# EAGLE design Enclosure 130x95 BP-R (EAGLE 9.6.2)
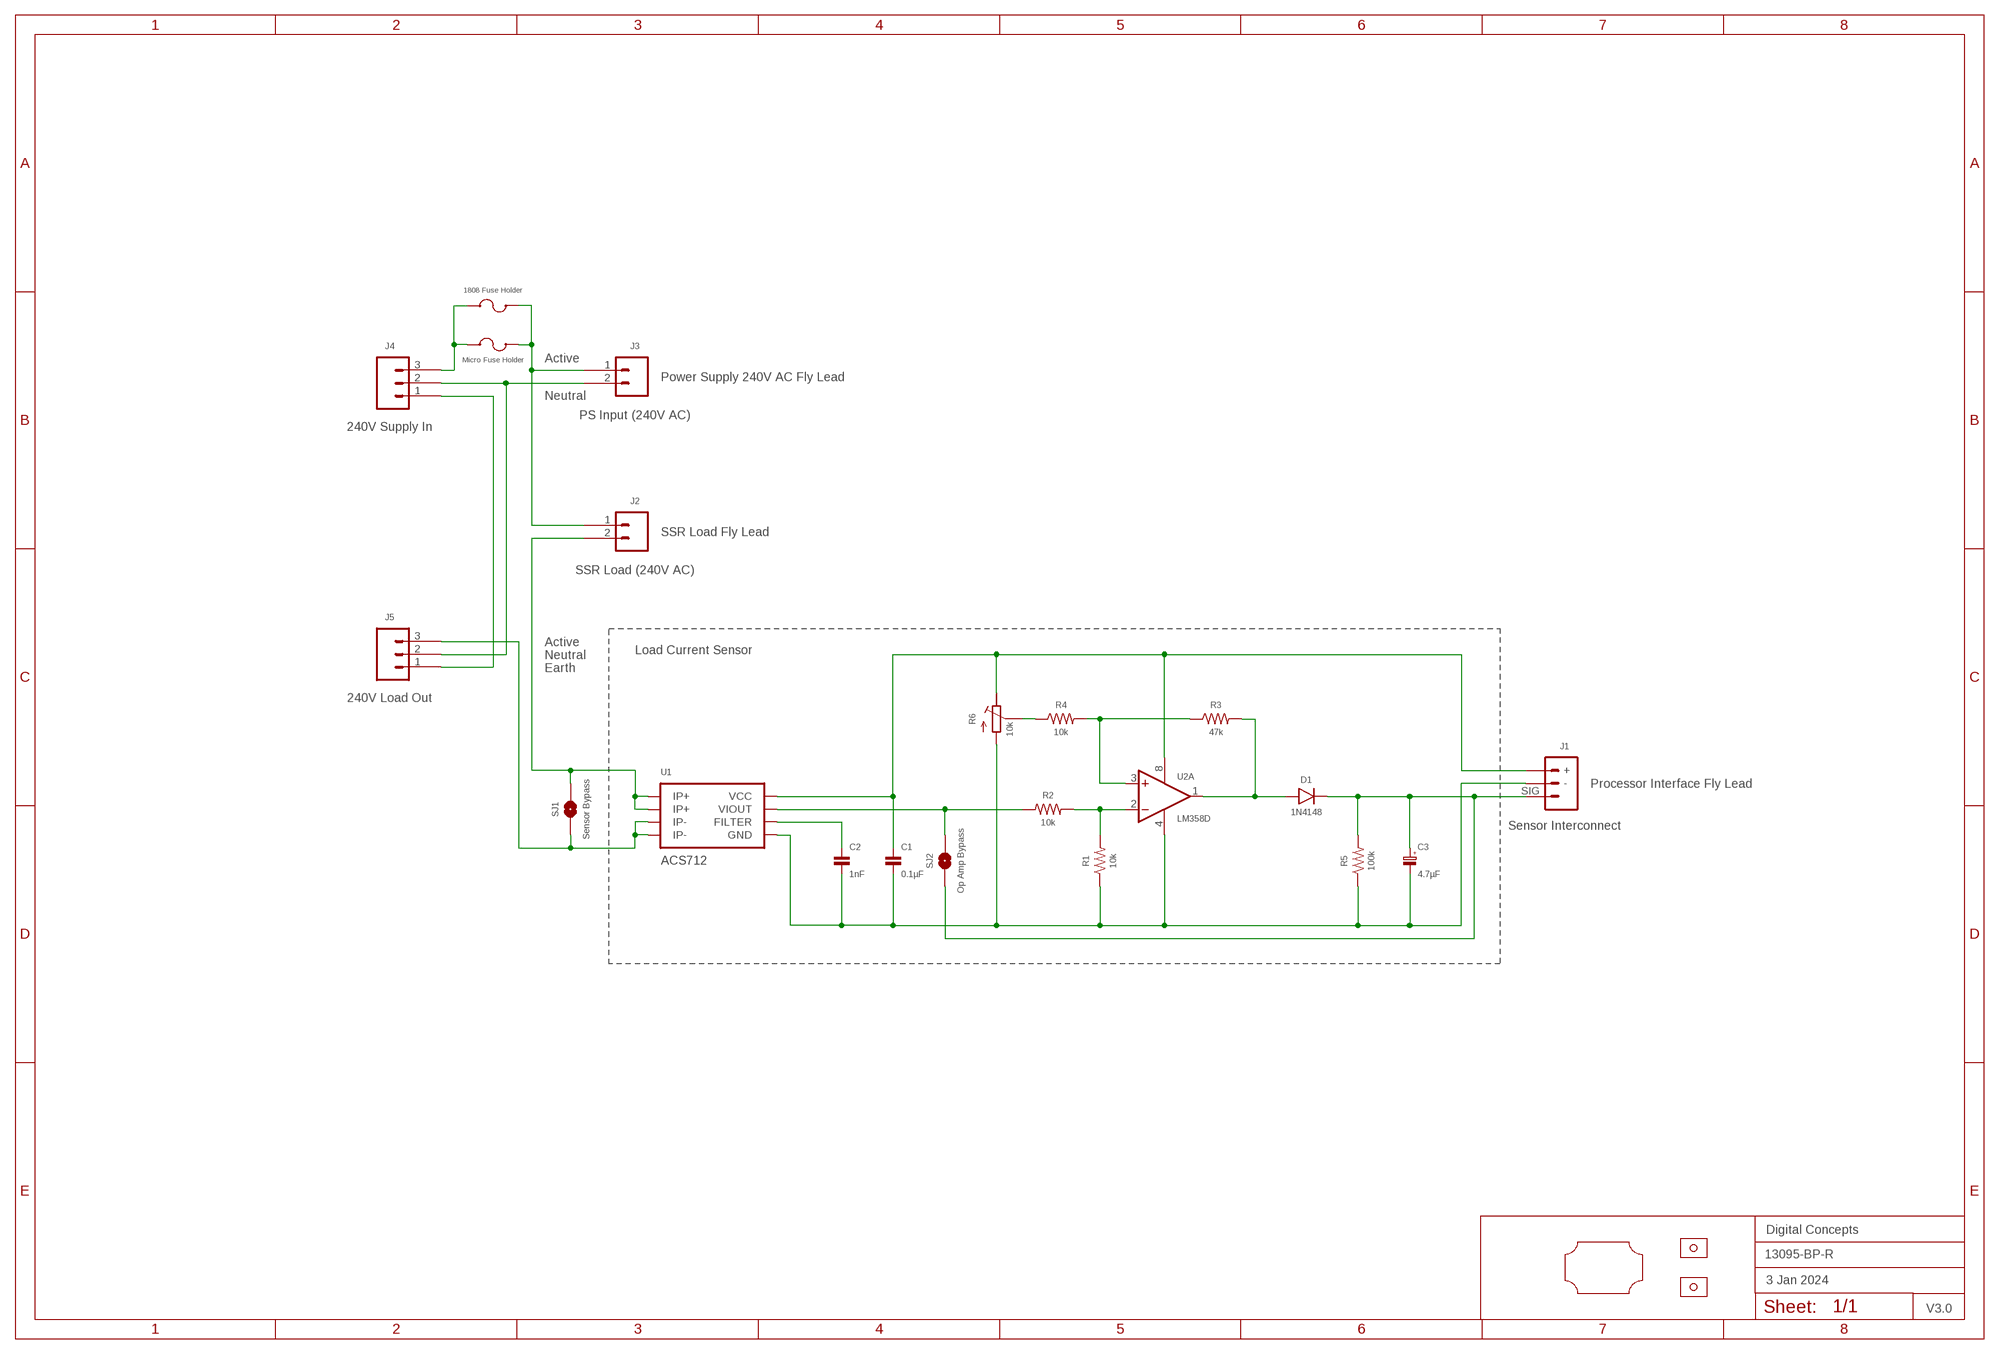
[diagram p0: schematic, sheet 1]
FRAME2 (A3L-LOC): DATE: 3 Jan 2024; OWNER: Digital Concepts; TITLE: 13095-BP-R; VERSION: V3.0

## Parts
C1  0.1µF  CAPACITOR-0805  [C0805]
C2  1nF  CAPACITOR-0805  [C0805]
C3  4.7µF  CAPACITOR-1206-TANTALUM  [C1206-POLARISED]
D1  1N4148  DIODE-1N4148-SOD323  [SOD-323]
F2  1808 Fuse Holder  FUSE-HOLDER-1808  [FUSE-HOLDER-1808]
J1  Sensor Interconnect  JST-PH2.0-3-HORIZONTAL  [JST-PH2.0-3-HORIZONTAL-SIG]
J2  SSR Load (240V AC)  TERMINAL_SCREW_2P_VERTICAL  [TERMINAL-SCREW-2P]
J3  PS Input (240V AC)  JST-XH2.54-2-HORIZONTAL  [JST-XH2.4-2-HORIZONTAL]
J4  240V Supply In  TERMINAL_SCREW_3P_VERTICAL  [TERMINAL-SCREW-3P]
J5  240V Load Out  TERMINAL_SCREW_3P_VERTICAL  [TERMINAL-SCREW-3P]
R1  10k  RESISTORR0805  [R0805]
R2  10k  RESISTORR0805  [R0805]
R3  47k  RESISTORR0805  [R0805]
R4  10k  RESISTORR0805  [R0805]
R5  100k  RESISTORR0805  [R0805]
R6  10k  RESISTOR-TRIMM-3386P  [RTRIM3386P]
SJ1  Sensor Bypass  SJ  [SJ]
SJ2  Op Amp Bypass  SJ  [SJ]
U1  ACS712  [SOP-8]
U2  LM358D  [SOP-8]
U$1  PCB-OUTLINE-130X95-MAX-RC-H3  [PROTO-130X95-OUTLINE-MAX-RC-H3]
U$2  Micro Fuse Holder  FUSE-HOLDER  [FUSE-HOLDER-MICRO]
U$4  STRAIN-RELIEF-SADDLE  [STRAIN-RELIEF-SADDLE]
U$5  STRAIN-RELIEF-SADDLE  [STRAIN-RELIEF-SADDLE]

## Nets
ACTIVE_IN: F2.P$2 J2.1 J3.1 U$2.P$3 U$2.P$4
ACTIVE_OUT: J2.2 SJ1.2 U1.1(IP+) U1.2(IP+)
EARTH: J4.1 J5.1
N$2: C1.1 J1.+ R6.1(E) U1.8(VCC) U2.8(P:V+)
N$3: C3.1(+) D1.C J1.SIG R5.2 SJ2.1
N$4: D1.A R3.2 U2.1(A:OUT)
N$5: R3.1 R4.2 U2.3(A:+IN)
N$6: R4.1 R6.2(S)
N$7: F2.P$1 J4.3 U$2.P$1 U$2.P$2
N$8: R1.2 R2.2 U2.2(A:-IN)
N$19: J5.3 SJ1.1 U1.3(IP-) U1.4(IP-)
N$20: C1.2 C2.2 C3.2(-) J1.- R1.1 R5.1 R6.3(A) U1.5(GND) U2.4(P:V-)
N$22: R2.1 SJ2.2 U1.7(VIOUT)
N$24: C2.1 U1.6(FILTER)
NEUTRAL: J3.2 J4.2 J5.2
Unconnected: U2.5(B:+IN) U2.6(B:-IN) U2.7(B:OUT)

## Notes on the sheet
- Active
- Power Supply 240V AC Fly Lead
- Neutral
- SSR Load Fly Lead
- Active
- Neutral | Load Current Sensor
- Earth
- Processor Interface Fly Lead

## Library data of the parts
C1 C2 = digitalconcepts:CAPACITOR-0805: 0805 Capacitor
C3 = digitalconcepts:CAPACITOR-1206-TANTALUM: Capacitor 1206 Tantalum
D1 = digitalconcepts:DIODE-1N4148-SOD323: 1N4148 SOD-323
F2 = digitalconcepts:FUSE-HOLDER-1808: 1808 Fuse Holder
J1 = digitalconcepts:JST-PH2.0-3-HORIZONTAL: PH2.0 3P Horizontal Connector
J2 = digitalconcepts:TERMINAL_SCREW_2P_VERTICAL: PCB Mount Screw-Type Terminal 2P
J3 = digitalconcepts:JST-XH2.54-2-HORIZONTAL: XH2.54 2P Horizontal Connector
J4 J5 = digitalconcepts:TERMINAL_SCREW_3P_VERTICAL: PCB Mount Screw-Type Terminal 3P
R1-R5 = digitalconcepts:RESISTOR: Resistor; SPICEPREFIX: R
R6 = digitalconcepts:RESISTOR-TRIMM-3386P: BOURNS Trim Pot 3386P
SJ1 SJ2 = digitalconcepts:SJ: Solder Jumper
U1 = digitalconcepts:ACS712: ACS712 Hall-Effect-Based Linear Current Sensor IC
U2 = digitalconcepts:LM358: OP AMP also LM158; LM258; LM2904 Source: http://cache.national.com/ds/LM/LM158.pdf
U$1 = digitalconcepts:PCB-OUTLINE-130X95-MAX-RC-H3: PCB Eagle Max-Right-Cropped outline for 130 x 95 enclosure (Horizontal format)
U$2 = digitalconcepts:FUSE-HOLDER: Fuse Holder
U$4 U$5 = digitalconcepts:STRAIN-RELIEF-SADDLE: Strain Relief Saddle (7mm x 13mm)

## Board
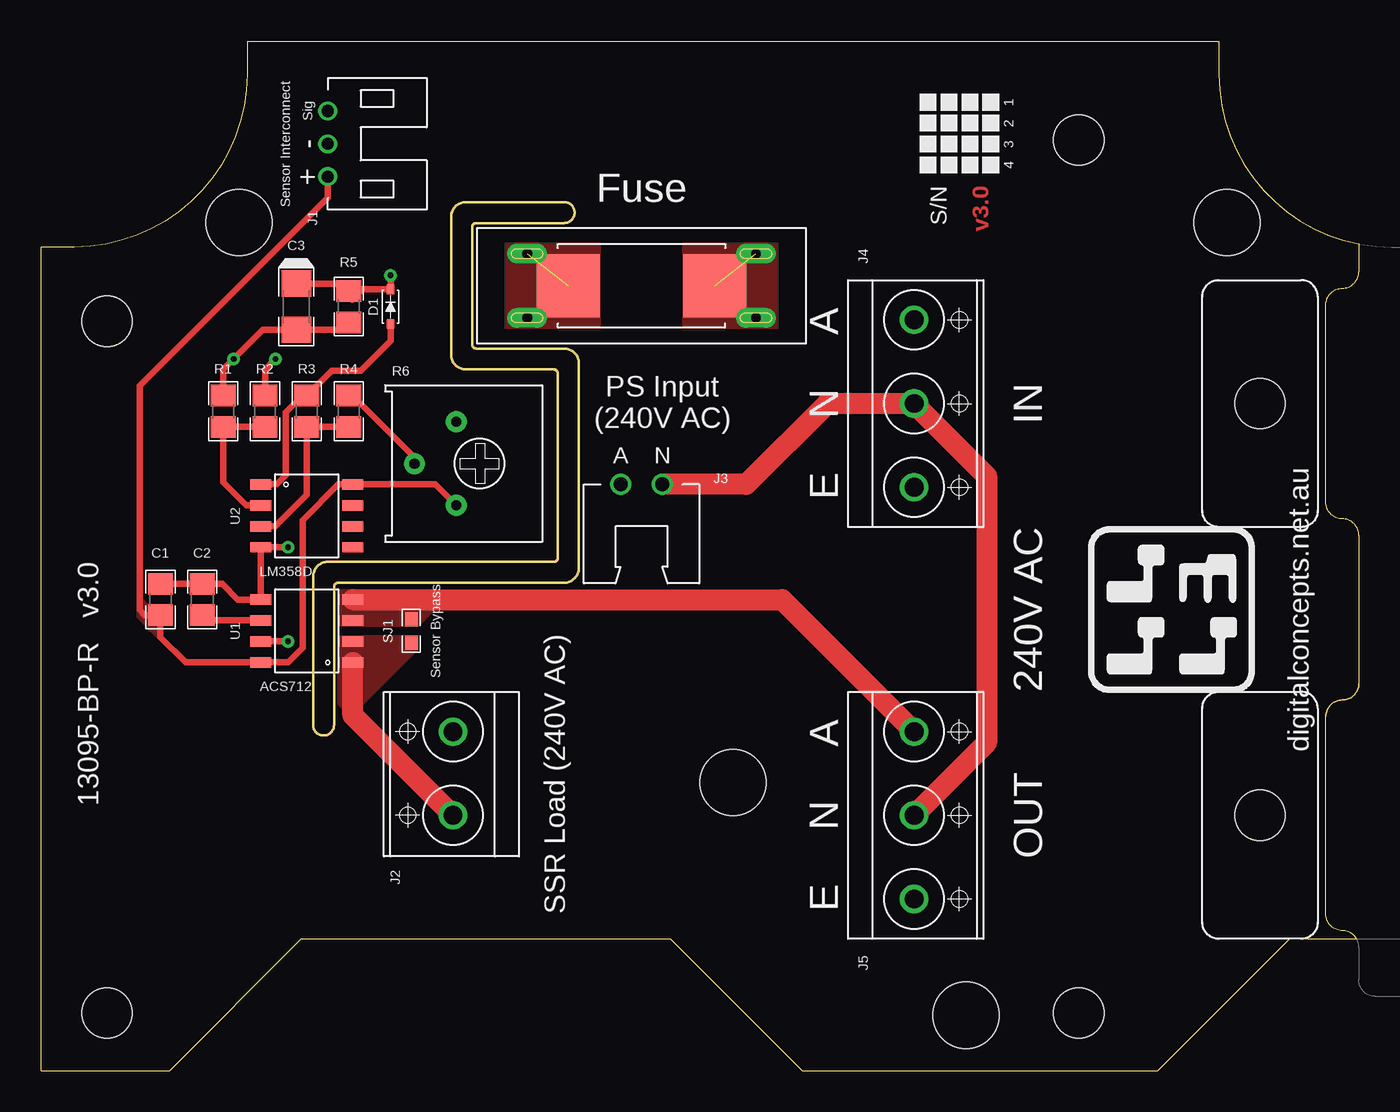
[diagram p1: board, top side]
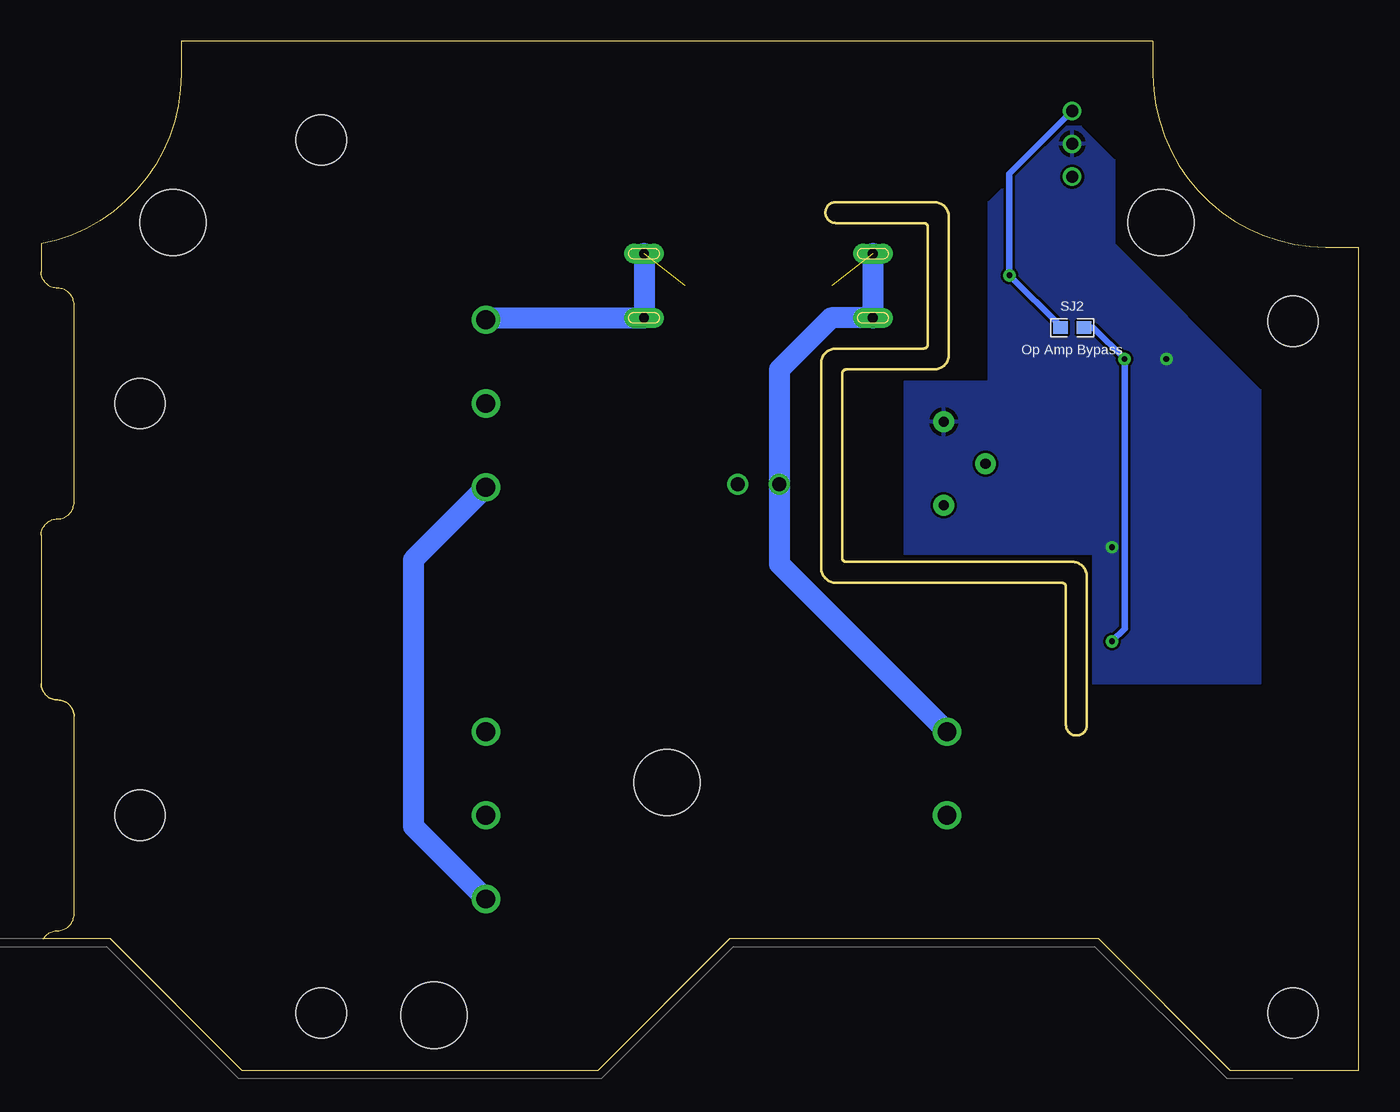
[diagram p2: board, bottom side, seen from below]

Size 80 x 62.5 mm. Coordinates in mm from the lower left corner, seen from the top.
Copper layers (1*16): Top 0.035mm / dielectric 1.5mm / Bottom 0.035mm
Design rules "default *": minimum track width 6mil, minimum drill 0.35mm, track to track 6mil, track to pad 6mil, pad to pad 6mil, via to via 6mil, smd to smd 6mil, copper to edge 6mil, drill to drill 6mil, minimum pad ring 1mil, minimum via ring 8mil, stop-mask expansion 4mil, vias tented up to drill 0mil, thermal gap 10mil
Milling: 24 lines

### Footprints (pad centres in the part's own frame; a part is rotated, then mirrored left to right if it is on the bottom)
C0805 = smd 1.3 x 1.5: 1 -0.95,0; 2 0.95,0
C1206-POLARISED = smd 1.6 x 1.8: 1 -1.4,0; 2 1.4,0
SOD-323 = smd 0.59 x 0.45: A -1.055,0; C 1.055,0
FUSE-HOLDER-1808 = smd 3.81 x 3.81: P$1 -4.445,0; P$2 4.445,0
JST-PH2.0-3-HORIZONTAL-SIG = drill 0.75: + 2,0; - 0,0; SIG -2,0
TERMINAL-SCREW-2P = drill 1.143: 1 -2.58,0; 2 2.5,0
JST-XH2.4-2-HORIZONTAL = drill 0.85: 1 1.27,0; 2 -1.27,0
TERMINAL-SCREW-3P = drill 1.143: 1 -5.08,0; 2 0,0; 3 5.08,0
R0805 = smd 1.3 x 1.5: 1 -0.95,0; 2 0.95,0
RTRIM3386P = drill 0.61 pad 1.27: 1 2.54,-0.45; 2 0,-2.99; 3 -2.54,-0.45
SJ = smd 0.864 x 0.762: 1 -0.711,0; 2 0.711,0
SOP-8 = smd 0.635 x 1.27: 1 -1.905,-2.794; 2 -0.635,-2.794; 3 0.635,-2.794; 4 1.905,-2.794; 5 1.905,2.794; 6 0.635,2.794; 7 -0.635,2.794; 8 -1.905,2.794
PROTO-130X95-OUTLINE-MAX-RC-H3 = hole 3.048: -38,10; 21,21; 21,-32; -38,-32 | hole 4: 0,-18; -30,16; 30,16; 14.14,-32.14
FUSE-HOLDER-MICRO = drill 0.6 pad 1.2 long: P$1 -6.95,1.95; P$2 -6.95,-1.95; P$3 6.95,-1.95; P$4 6.95,1.95
STRAIN-RELIEF-SADDLE = hole 3.048: 0,0

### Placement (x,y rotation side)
C1  7.24,28.6 90 top
C2  9.78,28.6 90 top
C3  15.5,46.38 270 top
D1  21.21,46.38 90 top
F2  36.45,47.65 180 top
J1  17.4,56.27 270 top
J2  25,18 270 top
J3  36.45,35.59 180 top
J4  53,40.5 90 top
J5  53,15.5 90 top
R1  11.05,40.03 270 top
R2  13.59,40.03 270 top
R3  16.13,40.03 90 top
R4  18.67,40.03 270 top
R5  18.67,46.38 90 top
R6  25.66,36.85 270 top
SJ1  22.48,26.7 270 top
SJ2  17.4,45.11 0 bottom
U1  16.13,26.7 90 top
U2  16.13,33.68 270 top
U$1  42,35.5 0 top
U$2  36.45,47.65 180 top
U$4  74,40.5 90 top
U$5  74,15.5 90 top

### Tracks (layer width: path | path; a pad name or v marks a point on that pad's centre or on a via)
ACTIVE_IN  (1 unrouted)
  Bottom 1.27: J2.1 35.18,30.76 J3.1 35.18,42.56 32.04,45.7 U$2.P$4 U$2.P$3
  pour Top (no thermals): 28.2,50.19 33.91,50.19 33.91,45.11 28.2,45.11
ACTIVE_OUT
  Top 1.27: J2.2 18.93,21.57 U1.1
  pour Top (no thermals): 18.04,26.44 22.86,26.44 22.86,25.55 19.18,21.87 18.42,21.87 18.04,22.25
EARTH
  Bottom 1.27: J4.1 57.41,31.02 57.41,14.82 J5.1
N$2
  Top 0.406: J1.+ 17.4,53 5.97,41.57 5.97,27.97 6.29,27.65 C1.1 7.24,26.31 8.76,24.79 U1.8 14.99,24.79 15.88,25.68 15.88,33.43 18.04,35.59 U2.8 23.93,35.59 R6.1
  pour Top (no thermals): 7.24,26.31 7.24,27.97 6.61,27.97 5.97,28.6 5.97,27.58
N$3  (via drill 0.35)
  Top 0.406: C3.1 18.22,47.78 R5.2 18.88,47.12 18.88,46.8 19.52,47.44 D1.C v21.21,48.28
  Bottom 0.406: J1.SIG 21.21,54.46 v21.21,48.28 18.11,45.19 SJ2.1
N$4
  Top 0.406: U2.1 14.29,35.59 14.86,36.15 14.86,39.96 15.88,40.98 R3.2 17.65,42.5 19.41,42.5 21.21,44.31 D1.A
N$5
  Top 0.406: U2.3 14.23,33.05 16.13,34.95 R3.1 R4.2
N$6
  Top 0.406: R6.2 22.66,37.24 18.92,40.98 R4.1
N$7  (1 unrouted)
  Bottom 1.27: U$2.P$2 U$2.P$1 52.88,45.7 J4.3
  pour Top (no thermals): 38.99,50.19 44.7,50.19 44.7,45.11 38.99,45.11
N$8
  Top 0.406: U2.2 12.45,34.31 11.05,35.71 R1.2 R2.2
N$19
  Top 1.27: J5.3 44.98,28.6 U1.4
  pour Top (no thermals): 18.04,29.23 23.75,29.23 24.38,28.6 24.38,28.47 22.86,26.95 18.04,26.95
N$20  (via drill 0.35)
  Top 0.406: C1.2 C2.2 10.99,29.55 11.94,28.6 U1.5 13.33,31.58 U2.4 v14.99,31.77 | R5.1 18.22,44.98 C3.2 13.46,44.98 v11.68,43.2 11.05,42.57 R1.1
  pour Bottom: 17.91,57.3 16.89,57.3 14.86,55.27 14.86,50.19 5.97,41.3 5.97,23.52 16.13,23.52 16.13,31.39 27.56,31.39 27.56,41.81 22.48,41.81 22.48,52.73
N$22  (via drill 0.35)
  Top 0.406: v14.23,43.2 13.59,42.57 R2.1 | v14.99,26.06 U1.7
  Bottom 0.406: v14.99,26.06 14.23,26.82 v14.23,43.2 16.13,45.11 SJ2.2
N$24
  Top 0.406: U1.6 10.1,27.33 C2.1
NEUTRAL
  Top 1.27: J3.2 42.8,35.59 47.72,40.5 J4.2 57.41,36.09 57.41,19.91 J5.2

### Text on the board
Top: v3.0
tPlace: 1 | 2 | 3 | 4 | S/N | digitalconcepts.net.au | 13095-BP-R v3.0
tNames: Fuse | A | N | IN | PS Input / (240V AC) | A | N | E | 240V AC | A | N | OUT | E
